[IBIS Ver]   3.2
[File Name]   sprm147.ibs
[File Rev]   0.0
[Date]   Nov 24, 2003
[Source]   File Originated at Texas Instruments
[Disclaimer]   Please be aware that in the absence of a written agreement
|   Texas Instruments(TI) assumes no liability for:
|   (1) The accuracy of the IBIS models provided to your company
|   (2) The proper functioning of these Models in your design
|   or for any resulting applications;or
|   (3) Infringement of patents,copyrights, or intellectual
|   property rights resulting from your use of these models.
|   TI provides IBIS Models as a service to our customers and
|   therefore reserves the right to limit distribution of the
|   Models.
[Copyright]   Property of Texas Instruments Incorporated.
|   Unauthorized reproduction and/or distribution is strictly
|   prohibited.
|   This product is protected under copyright law and trade
|   secret law as an unpublished work.
|   Created 1999,(C) Copyright 1999-2000,
|   Texas Instruments Incorporated., All Rights Reserved.
|   These commodities are under the U.S.
|   Government distribution license control.As such,they are not
|   to be re-exported without the prior approval of the U.S.
|   Department of Commerce.
[Notes]   Includes package and IO buffer models for 320c6416TGLZ7.
[Component]   c6416t_GLZ
[Manufacturer]   Texas Instruments
[Package]
|Variable   Typ   Min   Max
R_pkg   2.212e-01   1.101e-01   3.279e-01
L_pkg   4.011e-09   2.375e-09   5.798e-09
C_pkg   6.351e-13   3.910e-13   9.306e-13
[Pin] signal_name   model_name   R_pin   L_pin   C_pin
| Clock/PLL Configuration Section
   H4   CLKIN   IT33THYPD   1.801e-01   3.100e-09   6.130e-13
  AE6   CLKOUT4_GP1   BT3325ETPD   2.381e-01   4.630e-09   6.473e-13
  AD6   CLKOUT6_GP2   BT3325ETPD   2.343e-01   3.341e-09   7.539e-13
   G1   CLKMODE1   IT33TPD   2.962e-01   5.034e-09   7.789e-13
   H2   CLKMODE0   IT33THYPD   2.283e-01   3.995e-09   6.603e-13
| JTAG Emulation Section
 AB16   TMS   IT33THYPU   1.377e-01   2.655e-09   4.925e-13
 AE19   TDO   BT3350DTHYPU   2.511e-01   4.874e-09   6.498e-13
 AF18   TDI   IT33THYPU   2.614e-01   5.224e-09   6.920e-13
 AF16   TCLK   IT33THYPU   2.614e-01   5.224e-09   6.920e-13
 AB15   nTRST   IT33THYPD   2.614e-01   5.224e-09   6.920e-13
 AE18   EMU9   BT3325ETPU  2.477e-01   4.401e-09   6.871e-13
 AC17   EMU8   BT3325ETPU  1.709e-01   3.536e-09   5.334e-13
 AF17   EMU7   BT3325ETPU  2.500e-01   5.062e-09   6.512e-13
 AD17   EMU6   BT3325ETPU  1.890e-01   3.826e-09   4.936e-13
 AE17   EMU5   BT3325ETPU  2.341e-01   4.430e-09   6.507e-13
 AC16   EMU4   BT3325ETPU  1.551e-01   2.968e-09   5.512e-13
 AD16   EMU3   BT3325ETPU  1.987e-01   3.671e-09   6.373e-13
 AE16   EMU2   BT3325ETPU  2.124e-01   3.853e-09   6.090e-13
 AC15   EMU1   BT3325ETPU  1.646e-01   3.085e-09   5.799e-13
 AF15   EMU0   BT3325ETPU  2.591e-01   4.625e-09   6.938e-13
 AC18   EMU11   BT3325ETPU  1.860e-01   3.449e-09   5.618e-13
 AD18   EMU10   BT3325ETPU  2.025e-01   3.878e-09   5.902e-13
| Resets, Interrupts, and General-Purpose IOs
  AC7   nRESET   IT33THY   2.025e-01   3.878e-09   5.902e-13
   B4   NMI   IT33THYPD   2.697e-01   4.485e-09   7.472e-13
  AF4   GP7_EXTINT7   BT3350DTHYPU   2.697e-01   4.485e-09   7.472e-13
  AD5   GP6_EXTINT6   BT3350DTHYPU   2.697e-01   4.485e-09   7.472e-13
  AE5   GP5_EXTINT5   BT3350DTHYPU   2.697e-01   4.485e-09   7.472e-13
  AF5   GP4_EXTINT4   BT3350DTHYPU   2.697e-01   4.485e-09   7.472e-13
   G3   GP15_nPRST   BPCI66T   2.697e-01   4.485e-09   7.472e-13
   F2   GP14_PCLK   BPCI66T   2.546e-01   4.449e-09   7.097e-13
   G4   GP13_nPINTA   BPCI66T   2.546e-01   4.449e-09   7.097e-13
   J3   GP12_nPGNT   BPCI66T   2.546e-01   4.449e-09   7.097e-13
   F1   GP11_nPREQ   BPCI66T   2.546e-01   4.449e-09   7.097e-13
   L2   GP10_nPCBE3   BPCI66T   2.546e-01   4.449e-09   7.097e-13
   M3   GP9_PIDSEL   BPCI66T   1.917e-01   3.882e-09   5.354e-13
  AC6   GP3   BT3350CTHYPD   1.851e-01   3.359e-09   6.075e-13
  AF6   GP0   BT3350CTHYPD   2.922e-01   4.494e-09   8.253e-13
| Host-Port Interface (HPI) and Peripheral Component Interconnect (PCI)
  AA4   PCIEN   IT33THYPD   2.922e-01   4.494e-09   8.253e-13
   R4   nHINT_nPFRAME   BPCI66T   2.922e-01   4.494e-09   8.253e-13
   R1   HCNTL1_nPDEVSEL   BPCI66T   2.602e-01   4.276e-09   7.238e-13
   T4   HCNTL0_nPSTOP   BPCI66T   1.544e-01   3.008e-09   5.439e-13
   R3   HHWIL_nPTRDY   BPCI66T   1.544e-01   3.008e-09   5.439e-13
   P1   HR/nW_nPCBE2   BPCI66T   1.544e-01   3.008e-09   5.439e-13
   T3   nHAS_PPAR   BPCI66T   1.544e-01   3.008e-09   5.439e-13
   R2   nHCS_nPPERR   BPCI66T   1.544e-01   3.008e-09   5.439e-13
   T1   nHDS1_nPSERR   BPCI66T   1.544e-01   3.008e-09   5.439e-13
   T2   nHDS2_nPCBE1   BPCI66T   1.544e-01   3.008e-09   5.439e-13
   P4   nHRDY_nPIRDY   BPCI66T   1.432e-01   2.812e-09   4.868e-13
   J2   HD31_AD31   BPCI66T   2.239e-01   3.881e-09   6.413e-13
   K3   HD30_AD30   BPCI66T   2.011e-01   3.696e-09   5.567e-13
   J1   HD29_AD29   BPCI66T   2.725e-01   4.920e-09   7.166e-13
   K4   HD28_AD28   BPCI66T   1.590e-01   3.038e-09   5.268e-13
   K2   HD27_AD27   BPCI66T   2.196e-01   4.083e-09   6.214e-13
   L3   HD26_AD26   BPCI66T   1.822e-01   3.378e-09   5.755e-13
   K1   HD25_AD25   BPCI66T   2.676e-01   5.238e-09   6.857e-13
   L4   HD24_AD24   BPCI66T   1.692e-01   3.003e-09   5.620e-13
   L1   HD23_AD23   BPCI66T   2.646e-01   4.791e-09   6.858e-13
   M4   HD22_AD22   BPCI66T   1.455e-01   2.797e-09   5.032e-13
   M2   HD21_AD21   BPCI66T   2.098e-01   3.830e-09   5.948e-13
   N4   HD20_AD20   BPCI66T   1.611e-01   2.974e-09   5.102e-13
   M1   HD19_AD19   BPCI66T   2.475e-01   4.493e-09   6.660e-13
   N5   HD18_AD18   BPCI66T   1.114e-01   2.452e-09   4.378e-13
   N1   HD17_AD17   BPCI66T   2.536e-01   4.462e-09   6.731e-13
   P5   HD16_AD16   BPCI66T   1.387e-01   2.604e-09   5.119e-13
   U4   HD15_AD15   BPCI66T   1.709e-01   3.367e-09   5.453e-13
   U1   HD14_AD14   BPCI66T   2.504e-01   4.977e-09   6.598e-13
   U3   HD13_AD13   BPCI66T   1.886e-01   3.777e-09   4.994e-13
   U2   HD12_AD12   BPCI66T   2.321e-01   4.441e-09   6.047e-13
   V4   HD11_AD11   BPCI66T   1.869e-01   3.381e-09   5.890e-13
   V1   HD10_AD10   BPCI66T   2.598e-01   5.197e-09   6.873e-13
   V3   HD09_AD09   BPCI66T   2.598e-01   5.197e-09   6.873e-13
   V2   HD08_AD08   BPCI66T   2.598e-01   5.197e-09   6.873e-13
   W2   HD07_AD07   BPCI66T   2.598e-01   5.197e-09   6.873e-13
   W4   HD06_AD06   BPCI66T   2.598e-01   5.197e-09   6.873e-13
   Y1   HD05_AD05   BPCI66T   2.598e-01   5.197e-09   6.873e-13
   Y3   HD04_AD04   BPCI66T   2.598e-01   5.197e-09   6.873e-13
   Y2   HD03_AD03   BPCI66T   2.598e-01   5.197e-09   6.873e-13
   Y4   HD02_AD02   BPCI66T   2.598e-01   5.197e-09   6.873e-13
  AA1   HD01_AD01   BPCI66T   2.598e-01   5.197e-09   6.873e-13
  AA3   HD00_AD00   BPCI66T   2.598e-01   5.197e-09   6.873e-13
   W3   nPCBE0   BPCI66T   2.598e-01   5.197e-09   6.873e-13
  AD1   XSPCS   BT3350CTHYPD   2.598e-01   5.197e-09   6.873e-13
| EMIF A Control Signals
  L26   nACE3   BT3325ETPU  2.598e-01   5.197e-09   6.873e-13
  K23   nACE2   BT3325ETPU  2.598e-01   5.197e-09   6.873e-13
  K24   nACE1   BT3325ETPU  2.598e-01   5.197e-09   6.873e-13
  K25   nACE0   BT3325ETPU  2.598e-01   5.197e-09   6.873e-13
  T23   nABE07   BT3325ETPU  2.598e-01   5.197e-09   6.873e-13
  T24   nABE06   BT3325ETPU  2.598e-01   5.197e-09   6.873e-13
  R25   nABE05   BT3325ETPU  2.598e-01   5.197e-09   6.873e-13
  R26   nABE04   BT3325ETPU  2.598e-01   5.197e-09   6.873e-13
  M25   nABE03   BT3325ETPU  2.598e-01   5.197e-09   6.873e-13
  M26   nABE02   BT3325ETPU  2.598e-01   5.197e-09   6.873e-13
  L23   nABE01   BT3325ETPU  2.598e-01   5.197e-09   6.873e-13
  L24   nABE00   BT3325ETPU  2.598e-01   5.197e-09   6.873e-13
  M22   nAPDT   BT3325ETPU  2.598e-01   5.197e-09   6.873e-13
| EMIF A Bus Arbitration
  N22   nAHOLDA   BT3325ETPU  2.598e-01   5.197e-09   6.873e-13
  V23   nAHOLD   IT33THYPU   2.598e-01 5.197e-09   6.873e-13
  P22   ABUSREQ0   BT3325ETPU  2.598e-01   5.197e-09   6.873e-13
| EMIF A Async/Sync Memory Control
  H25   AECLKIN   IT33THYPD   2.511e-01 4.592e-09   6.768e-13
  J23   AECLKOUT2   BT3325ETPD  1.851e-01   3.434e-09   5.608e-13
  J26   AECLKOUT1   BT3325ETPD  2.599e-01   5.229e-09   6.780e-13
  J25   nASDCAS   BT3325ETPU  2.467e-01   4.341e-09   6.879e-13
  J24   nASDRAS   BT3325ETPU  2.014e-01   3.844e-09   5.854e-13
  K26   nASDWE   BT3325ETPU  2.494e-01   5.112e-09   6.385e-13
  L25   ASDCKE   BT3325ETPU  2.118e-01   3.884e-09   5.955e-13
  R22   nASOE3   BT3325ETPU  2.118e-01   3.884e-09   5.955e-13
  L22   AARDY   IT33THYPU   1.370e-01 2.710e-09   4.841e-13
| EMIF A Address
  T22   AEA22   BT3325ETPD  1.229e-01   2.684e-09   4.276e-13
  V24   AEA21   BT3325ETPD  2.064e-01   3.768e-09   6.312e-13
  V25   AEA20   BT3325ETPD  2.195e-01   4.186e-09   6.132e-13
  V26   AEA19   BT3325ETPD  2.732e-01   4.782e-09   7.055e-13
  U23   AEA18   BT3325ETPD  1.584e-01   2.852e-09   5.393e-13
  U24   AEA17   BT3325ETPD  2.008e-01   3.829e-09   5.212e-13
  U25   AEA16   BT3325ETPD  2.141e-01   4.207e-09   5.706e-13
  U26   AEA15   BT3325ETPD  2.663e-01   5.219e-09   6.884e-13
  T25   AEA14   BT3325ETPD  2.291e-01   3.977e-09   6.514e-13
  T26   AEA13   BT3325ETPD  2.614e-01   4.919e-09   6.730e-13
  R23   AEA12   BT3325ETPD  1.480e-01   3.031e-09   5.090e-13
  R24   AEA11   BT3325ETPD  1.952e-01   3.745e-09   6.090e-13
  P23   AEA10   BT3325ETPD  1.599e-01   3.076e-09   4.973e-13
  P24   AEA09   BT3325ETPD  1.599e-01   3.076e-09   4.973e-13
  P26   AEA08   BT3325ETPD  1.599e-01   3.076e-09   4.973e-13
  N23   AEA07   BT3325ETPD  1.599e-01   3.076e-09   4.973e-13
  N24   AEA06   BT3325ETPD  1.599e-01   3.076e-09   4.973e-13
  N26   AEA05   BT3325ETPD  1.599e-01   3.076e-09   4.973e-13
  M23   AEA04   BT3325ETPD  1.599e-01   3.076e-09   4.973e-13
  M24   AEA03   BT3325ETPD  1.599e-01   3.076e-09   4.973e-13
| EMIF A Data
 AF24   AED63   BT3325ETPU  3.137e-01   4.620e-09   8.662e-13
 AF23   AED62   BT3325ETPU  3.279e-01   4.771e-09   9.306e-13
 AE23   AED61   BT3325ETPU  2.711e-01   4.106e-09   8.091e-13
 AE22   AED60   BT3325ETPU  2.891e-01   4.209e-09   8.615e-13
 AD22   AED59   BT3325ETPU  2.423e-01   3.976e-09   6.864e-13
 AF22   AED58   BT3325ETPU  2.977e-01   4.773e-09   8.420e-13
 AD21   AED57   BT3325ETPU  2.300e-01   3.370e-09   7.485e-13
 AE21   AED56   BT3325ETPU  2.753e-01   4.129e-09   8.309e-13
 AC21   AED55   BT3325ETPU  2.164e-01   3.287e-09   6.853e-13
 AF21   AED54   BT3325ETPU  2.835e-01   5.063e-09   7.235e-13
 AD20   AED53   BT3325ETPU  2.224e-01   4.053e-09   6.338e-13
 AE20   AED52   BT3325ETPU  2.582e-01   4.676e-09   6.914e-13
 AC20   AED51   BT3325ETPU  2.074e-01   3.082e-09   7.302e-13
 AF20   AED50   BT3325ETPU  2.708e-01   4.795e-09   7.375e-13
 AC19   AED49   BT3325ETPU  1.905e-01   3.252e-09   6.365e-13
 AD19   AED48   BT3325ETPU  2.081e-01   3.848e-09   5.927e-13
  W24   AED47   BT3325ETPU  2.123e-01   3.951e-09   6.323e-13
  W23   AED46   BT3325ETPU  1.710e-01   3.189e-09   5.673e-13
  Y26   AED45   BT3325ETPU  2.823e-01   4.619e-09   7.521e-13
  Y23   AED44   BT3325ETPU  1.758e-01   3.461e-09   5.750e-13
  Y25   AED43   BT3325ETPU  2.336e-01   4.207e-09   6.577e-13
  Y24   AED42   BT3325ETPU  2.187e-01   3.908e-09   6.476e-13
 AA26   AED41   BT3325ETPU  2.881e-01   5.195e-09   7.377e-13
 AA23   AED40   BT3325ETPU  1.857e-01   3.342e-09   6.147e-13
 AA25   AED39   BT3325ETPU  2.386e-01   4.607e-09   6.579e-13
 AA24   AED38   BT3325ETPU  2.252e-01   4.506e-09   5.857e-13
 AB26   AED37   BT3325ETPU  3.007e-01   5.253e-09   7.746e-13
 AB24   AED36   BT3325ETPU  2.392e-01   4.041e-09   6.955e-13
 AB25   AED35   BT3325ETPU  2.521e-01   4.603e-09   6.570e-13
 AC25   AED34   BT3325ETPU  2.807e-01   4.863e-09   7.510e-13
 AC26   AED33   BT3325ETPU  2.960e-01   5.121e-09   7.683e-13
 AD26   AED32   BT3325ETPU  3.008e-01   4.916e-09   8.215e-13
  C26   AED31   BT3325ETPU  3.097e-01   5.406e-09   7.617e-13
  D26   AED30   BT3325ETPU  3.225e-01   5.517e-09   8.165e-13
  D25   AED29   BT3325ETPU  2.683e-01   4.604e-09   7.287e-13
  E25   AED28   BT3325ETPU  2.825e-01   4.968e-09   7.318e-13
  E24   AED27   BT3325ETPU  2.414e-01   4.280e-09   6.457e-13
  E26   AED26   BT3325ETPU  2.953e-01   5.146e-09   7.737e-13
  F24   AED25   BT3325ETPU  2.271e-01   4.100e-09   5.755e-13
  F25   AED24   BT3325ETPU  2.711e-01   4.743e-09   7.222e-13
  F23   AED23   BT3325ETPU  2.131e-01   3.580e-09   6.337e-13
  F26   AED22   BT3325ETPU  2.841e-01   5.079e-09   7.359e-13
  G24   AED21   BT3325ETPU  2.217e-01   4.037e-09   6.338e-13
  G25   AED20   BT3325ETPU  2.556e-01   4.841e-09   6.769e-13
  G23   AED19   BT3325ETPU  2.034e-01   3.544e-09   6.297e-13
  G26   AED18   BT3325ETPU  2.698e-01   4.780e-09   7.327e-13
  H23   AED17   BT3325ETPU  1.904e-01   3.427e-09   5.839e-13
  H24   AED16   BT3325ETPU  2.066e-01   3.899e-09   5.834e-13
  C19   AED15   BT3325ETPU  2.140e-01   3.969e-09   6.377e-13
  D19   AED14   BT3325ETPU  1.703e-01   3.235e-09   5.662e-13
  A20   AED13   BT3325ETPU  2.811e-01   4.710e-09   7.445e-13
  D20   AED12   BT3325ETPU  1.756e-01   3.477e-09   5.767e-13
  B20   AED11   BT3325ETPU  2.338e-01   4.170e-09   6.537e-13
  C20   AED10   BT3325ETPU  2.189e-01   3.889e-09   6.502e-13
  A21   AED09   BT3325ETPU  2.189e-01   3.889e-09   6.502e-13
  D21   AED08   BT3325ETPU  2.189e-01   3.889e-09   6.502e-13
  B21   AED07   BT3325ETPU  2.189e-01   3.889e-09   6.502e-13
  C21   AED06   BT3325ETPU  2.189e-01   3.889e-09   6.502e-13
  A22   AED05   BT3325ETPU  2.189e-01   3.889e-09   6.502e-13
  C22   AED04   BT3325ETPU  2.189e-01   3.889e-09   6.502e-13
  B22   AED03   BT3325ETPU  2.189e-01   3.889e-09   6.502e-13
  B23   AED02   BT3325ETPU  2.189e-01   3.889e-09   6.502e-13
  A23   AED01   BT3325ETPU  2.189e-01   3.889e-09   6.502e-13
  A24   AED00   BT3325ETPU  2.189e-01   3.889e-09   6.502e-13
| EMIF B Control Signals
  A13   nBCE3   BT3325ETPU  2.189e-01   3.889e-09   6.502e-13
  C12   nBCE2   BT3325ETPU  2.189e-01   3.889e-09   6.502e-13
  B12   nBCE1   BT3325ETPU  2.189e-01   3.889e-09   6.502e-13
  A12   nBCE0   BT3325ETPU  2.189e-01   3.889e-09   6.502e-13
  D13   nBBE01   BT3325ETPU  2.189e-01   3.889e-09   6.502e-13
  C13   nBBE00   BT3325ETPU  2.189e-01   3.889e-09   6.502e-13
  E12   nBPDT   BT3325ETPU  2.189e-01   3.889e-09   6.502e-13
| EMIF B Bus Arbitration
  E13   nBHOLDA   BT3325ETPU  2.189e-01   3.889e-09   6.502e-13
  B19   nBHOLD   IT33THYPU   2.189e-01   3.889e-09   6.502e-13
  E14   BBUSREQ0   BT3325ETPU  2.189e-01   3.889e-09   6.502e-13
| EMIF B Async/Sync Memory Control
  A11   BECLKIN   IT33THYPD   2.464e-01  4.786e-09   6.528e-13
  D11   BECLKOUT2   BT3325ETPD  1.551e-01   3.003e-09   5.234e-13
  D12   BECLKOUT1   BT3325ETPD  1.654e-01   3.214e-09   5.248e-13
  A10   nBSDCAS   BT3325ETPU  2.586e-01   5.225e-09   6.597e-13
  B11   nBSDRAS   BT3325ETPU  2.119e-01   3.872e-09   5.932e-13
  C11   nBSDWE   BT3325ETPU  1.986e-01   3.667e-09   5.913e-13
  E15   nBSOE3   BT3325ETPU  1.986e-01   3.667e-09   5.913e-13
  E11   BARDY   IT33THY   1.365e-01   2.770e-09   4.880e-13
| EMIF B Address
  E16   BEA20   BT3325ETPU  1.226e-01   2.604e-09   4.665e-13
  D18   BEA19   BT3325ETPU  1.641e-01   2.969e-09   5.594e-13
  C18   BEA18   BT3325ETPD  2.067e-01   3.758e-09   6.201e-13
  B18   BEA17   BT3325ETPD  2.194e-01   4.208e-09   6.099e-13
  A18   BEA16   BT3325ETPD  2.767e-01   5.325e-09   6.838e-13
  D17   BEA15   BT3325ETPD  1.577e-01   2.912e-09   5.360e-13
  C17   BEA14   BT3325ETPD  2.010e-01   3.803e-09   5.328e-13
  B17   BEA13   BT3325ETPD  2.141e-01   4.201e-09   5.714e-13
  A17   BEA12   BT3325ETPD  2.663e-01   5.209e-09   6.868e-13
  D16   BEA11   BT3325ETPD  1.659e-01   3.222e-09   5.785e-13
  C16   BEA10   BT3325ETPD  1.798e-01   3.385e-09   6.098e-13
  B16   BEA09   BT3325ETPD  1.798e-01   3.385e-09   6.098e-13
  A16   BEA08   BT3325ETPD  1.798e-01   3.385e-09   6.098e-13
  D15   BEA07   BT3325ETPD  1.798e-01   3.385e-09   6.098e-13
  C15   BEA06   BT3325ETPD  1.798e-01   3.385e-09   6.098e-13
  B15   BEA05   BT3325ETPD  1.798e-01   3.385e-09   6.098e-13
  A15   BEA04   BT3325ETPD  1.798e-01   3.385e-09   6.098e-13
  D14   BEA03   BT3325ETPD  1.798e-01   3.385e-09   6.098e-13
  C14   BEA02   BT3325ETPD  1.798e-01   3.385e-09   6.098e-13
  A14   BEA01   BT3325ETPD  1.798e-01   3.385e-09   6.098e-13
| EMIF B Data
   D7   BED15   BT3325ETPU  2.025e-01   3.629e-09   6.353e-13
   B6   BED14   BT3325ETPU  2.713e-01   4.736e-09   7.195e-13
   C7   BED13   BT3325ETPU  2.210e-01   4.136e-09   6.396e-13
   A6   BED12   BT3325ETPU  2.839e-01   5.035e-09   7.333e-13
   D8   BED11   BT3325ETPU  1.903e-01   3.261e-09   6.403e-13
   B7   BED10   BT3325ETPU  2.577e-01   4.650e-09   6.879e-13
   C8   BED09   BT3325ETPU  2.577e-01   4.650e-09   6.879e-13
   A7   BED08   BT3325ETPU  2.577e-01   4.650e-09   6.879e-13
   C9   BED07   BT3325ETPU  2.577e-01   4.650e-09   6.879e-13
   B8   BED06   BT3325ETPU  2.577e-01   4.650e-09   6.879e-13
   D9   BED05   BT3325ETPU  2.577e-01   4.650e-09   6.879e-13
   B9   BED04   BT3325ETPU  2.577e-01   4.650e-09   6.879e-13
  C10   BED03   BT3325ETPU  2.577e-01   4.650e-09   6.879e-13
   A9   BED02   BT3325ETPU  2.577e-01   4.650e-09   6.879e-13
  D10   BED01   BT3325ETPU  2.577e-01   4.650e-09   6.879e-13
  B10   BED00   BT3325ETPU  2.577e-01   4.650e-09   6.879e-13
| Timer 2
   A4   TOUT2   BT3350CTHYPD   3.211e-01   5.798e-09   7.928e-13
   C5   TINP2   IT33THYPD   2.423e-01  4.149e-09   6.777e-13
| Timer 1
   B5   TOUT1   BT3350CTHYPD   2.850e-01   4.720e-09   7.582e-13
   A5   TINP1   IT33THYPD   2.956e-01  5.023e-09   7.720e-13
| Timer 0
   D6   TOUT0   BT3350CTHYPD   2.113e-01   3.835e-09   6.281e-13
   C6   TINP0   IT33THYPD   2.266e-01  4.066e-09   6.171e-13
| MultiChannel Buffered Serial Port 2 (McBSP2)
  AF3   MCBSP2_EN   IT33THYPD   3.053e-01  4.791e-09   8.195e-13
  AE4   CLKS2_GP8   BT3350CTHYPD   2.815e-01   4.759e-09   7.525e-13
  AB1   CLKR2   BT3350CTHYPD   2.952e-01   5.337e-09   7.495e-13
  AC2   CLKX2_XSPCLK   BT3350CTHYPD   2.690e-01   4.510e-09   7.463e-13
  AB3   DR2_XSPDI   IT33TPU 2.430e-01   4.177e-09   6.584e-13
  AA2   DX2_XSPDO   BT3350DTHYPU   2.703e-01   4.736e-09   7.142e-13
  AC1   FSR2   BT3350CTHYPD   3.209e-01   5.708e-09   7.989e-13
  AB2   FSX2   BT3350CTHYPD   2.854e-01   4.677e-09   7.645e-13
| MultiChannel Buffered Serial Port 1 (McBSP1)
  AC8   CLKS1_URADDR3   BT3350DTHY  1.696e-01   3.371e-09   5.336e-13
 AC10   CLKR1_URADDR2   BT3350DTHY  1.577e-01   2.917e-09   5.345e-13
 AB12   CLKX1_URADDR4   BT3350DTHY  1.314e-01   2.568e-09   4.920e-13
 AF11   DR1_UXADDR1   BT3350DTHY  2.619e-01   4.872e-09   6.818e-13
 AB11   DX1_UXADDR4   BT3350DTHY  1.224e-01   2.641e-09   4.477e-13
  AC9   FSR1_UXADDR2   BT3350DTHY  1.641e-01   2.958e-09   5.482e-13
 AB13   FSX1_UXADDR3   BT3350DTHY  1.112e-01   2.390e-09   4.431e-13
| MultiChannel Buffered Serial Port 0 (McBSP0)
   F4   CLKS0   IT33THYPD   1.913e-01  3.477e-09   6.149e-13
   D1   CLKR0   BT3350CTHYPD   2.976e-01   5.157e-09   7.602e-13
   E1   CLKX0   BT3350CTHYPD   3.080e-01   5.297e-09   7.859e-13
   D2   DR0   IT33TPU 2.825e-01   4.838e-09   7.380e-13
   E2   DX0   BT3350DTHYPU   2.580e-01   4.588e-09   6.760e-13
   C1   FSR0   BT3350CTHYPD   3.009e-01   4.906e-09   7.948e-13
   E3   FSX0   BT3350CTHYPD   2.445e-01   4.090e-09   6.962e-13
| UTOPIA Transmit Interface
 AD11   UXCLK   IT33THY   1.796e-01   3.416e-09   5.747e-13
 AC14   UXCLAV   BT3350DTHY  1.451e-01   2.709e-09   4.991e-13
 AE15   nUXENB   BT3350DTHY  1.451e-01   2.709e-09   4.991e-13
 AC13   UXSOC   BT3350DTHY  1.609e-01   2.896e-09   5.178e-13
  AE9   UXADDR0   BT3350DTHY  2.212e-01   4.035e-09   6.442e-13
 AD10   UXDATA7   BT3350DTHY  2.009e-01   3.820e-09   5.217e-13
  AD9   UXDATA6   BT3350DTHY  2.069e-01   3.735e-09   6.102e-13
  AD8   UXDATA5   BT3350DTHY  2.137e-01   4.020e-09   6.080e-13
  AE8   UXDATA4   BT3350DTHY  2.278e-01   4.253e-09   6.349e-13
  AF9   UXDATA3   BT3350DTHY  2.793e-01   5.310e-09   6.864e-13
  AF7   UXDATA2   BT3350DTHY  2.810e-01   4.704e-09   7.582e-13
  AE7   UXDATA1   BT3350DTHY  2.331e-01   4.270e-09   6.513e-13
  AD7   UXDATA0   BT3350DTHY  2.198e-01   3.771e-09   6.554e-13
| UTOPIA Receive Interface
 AD12   URCLK   IT33THY   1.922e-01   3.803e-09   5.427e-13
 AF14   URCLAV   BT3350DTHY  2.495e-01   4.260e-09   6.591e-13
 AD15   nURENB   BT3350DTHY  2.495e-01   4.260e-09   6.591e-13
 AB14   URSOC   IT33T   1.337e-01   2.442e-09   4.893e-13
 AF10   URADDR1   BT3350DTHY  2.663e-01   5.227e-09   6.845e-13
 AE10   URADDR0   BT3350DTHY  2.146e-01   4.151e-09   5.705e-13
 AF12   URDATA7   IT33T   2.456e-01   4.323e-09   6.794e-13
 AE11   URDATA6   IT33T   2.291e-01   4.061e-09   6.408e-13
 AF13   URDATA5   IT33T   2.560e-01   4.376e-09   6.811e-13
 AC11   URDATA4   IT33T   1.656e-01   3.268e-09   5.357e-13
 AC12   URDATA3   IT33T   1.441e-01   3.075e-09   4.975e-13
 AE12   URDATA2   IT33T   2.104e-01   3.651e-09   6.043e-13
 AD14   URDATA1   IT33T   1.921e-01   3.213e-09   5.935e-13
 AD13   URDATA0   IT33T   1.677e-01   5.324e-09   3.910e-13
| End of Package Model
[Component]   IT33T
[Manufacturer]   Texas Instruments
[Package]
|   typ   min   max
R_pkg   0   0   0
L_pkg   0   0   0
C_pkg   0   0   0
[Pin]   signal_name   model_name   R_pin   L_pin   C_pin
   1   A   IT33T   0   0   0
[Component]   BT3325ETPD
[Manufacturer]   Texas Instruments
[Package]
|   typ   min   max
R_pkg   0   0   0
L_pkg   0   0   0
C_pkg   0   0   0
[Pin]   signal_name   model_name   R_pin   L_pin   C_pin
   1   Y   BT3325ETPD   0   0   0
[Component]   IT33TPU
[Manufacturer]   Texas Instruments
[Package]
|   typ   min   max
R_pkg   0   0   0
L_pkg   0   0   0
C_pkg   0   0   0
[Pin]   signal_name   model_name   R_pin   L_pin   C_pin
   1   A   IT33TPU   0   0   0
[Component]   BT3350DTHYPU
[Manufacturer]   Texas Instruments
[Package]
|   typ   min   max
R_pkg   0   0   0
L_pkg   0   0   0
C_pkg   0   0   0
[Pin]   signal_name   model_name   R_pin   L_pin   C_pin
   1   Y   BT3350DTHYPU   0   0   0
[Component]   BT3325ETPU
[Manufacturer]   Texas Instruments
[Package]
|   typ   min   max
R_pkg   0   0   0
L_pkg   0   0   0
C_pkg   0   0   0
[Pin]   signal_name   model_name   R_pin   L_pin   C_pin
   1   Y   BT3325ETPU   0   0   0
[Component]   IT33THY
[Manufacturer]   Texas Instruments
[Package]
|   typ   min   max
R_pkg   0   0   0
L_pkg   0   0   0
C_pkg   0   0   0
[Pin]   signal_name   model_name   R_pin   L_pin   C_pin
   1   A   IT33THY   0   0   0
[Component]   IT33THYPU
[Manufacturer]   Texas Instruments
[Package]
|   typ   min   max
R_pkg   0   0   0
L_pkg   0   0   0
C_pkg   0   0   0
[Pin]   signal_name   model_name   R_pin   L_pin   C_pin
   1   A   IT33THYPU   0   0   0
[Component]   IT33THYPD
[Manufacturer]   Texas Instruments
[Package]
|   typ   min   max
R_pkg   0   0   0
L_pkg   0   0   0
C_pkg   0   0   0
[Pin]   signal_name   model_name   R_pin   L_pin   C_pin
   1   A   IT33THYPD   0   0   0
[Component]   BPCI66T
[Manufacturer]   Texas Instruments
[Package]
|   typ   min   max
R_pkg   0   0   0
L_pkg   0   0   0
C_pkg   0   0   0
[Pin]   signal_name   model_name   R_pin   L_pin   C_pin
   1   Y   BPCI66T   0   0   0
[Component]   BT3350CTHYPD
[Manufacturer]   Texas Instruments
[Package]
|   typ   min   max
R_pkg   0   0   0
L_pkg   0   0   0
C_pkg   0   0   0
[Pin]   signal_name   model_name   R_pin   L_pin   C_pin
   1   Y   BT3350CTHYPD   0   0   0
[Component]   BT3350DTHY
[Manufacturer]   Texas Instruments
[Package]
|   typ   min   max
R_pkg   0   0   0
L_pkg   0   0   0
C_pkg   0   0   0
[Pin]   signal_name   model_name   R_pin   L_pin   C_pin
   1   Y   BT3350DTHY   0   0   0
[Component]   IT33TPD
[Manufacturer]   Texas Instruments
[Package]
|   typ   min   max
R_pkg   0   0   0
L_pkg   0   0   0
C_pkg   0   0   0
[Pin]   signal_name   model_name   R_pin   L_pin   C_pin
   1   A   IT33TPD   0   0   0
| Models and submodels in the file (12): IT33T (Input), BT3325ETPD (I/O), IT33TPU (Input), BT3350DTHYPU (I/O), BT3325ETPU (I/O), IT33THY (Input), IT33THYPU (Input), IT33THYPD (Input), BPCI66T (I/O), BT3350CTHYPD (I/O), BT3350DTHY (I/O), IT33TPD (Input)
